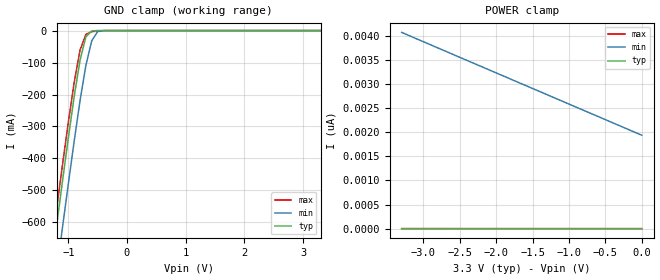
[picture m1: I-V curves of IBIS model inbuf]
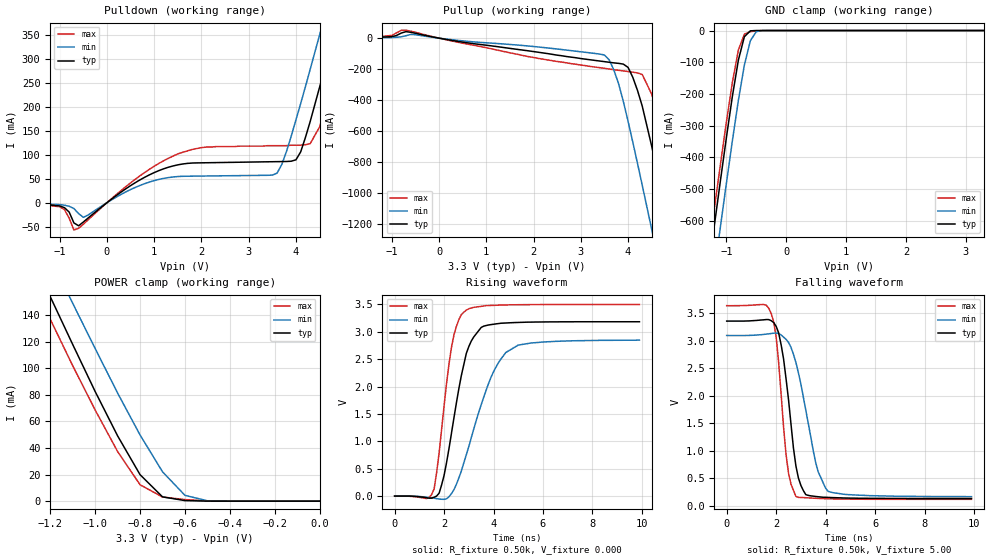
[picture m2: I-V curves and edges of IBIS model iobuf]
| IBIS file 43244k.ibs created by s2ibis2 version 1.0
| North Carolina State University Electronics Research Laboratory  1995
[IBIS ver]   2.1
[File name]   74fct3244.ibs
[File Rev]   0.1
[Date]   Wednesday, March 19, 1997
[Source]   IDT
[Notes]   1. Temp typ=25C, min=100C, max=0C 2. Ramp rates based on 500
   ohm load
[Copyright]   Copyright 1997, Integrated Device Technology, Inc.
|   Component IDT54/74FCT3245/A
[Component]   IDT54/74FCT3244/A
[Manufacturer]   Integrated Device Technology Inc.
[Package]
| Following package parameters are for D20-1(CDIP), P20-1(DPIP) packages
|[Package]
|| variable   typ   min   max
|R_pkg   40.00m   30.00m   50.00m
|L_pkg   7.00nH   4.00nH   10.00nH
|C_pkg   0.60pF   0.50pF   0.70pF
| Following package parameters are for SO20-6(EIAJ), SO20-2(SOIC) packages
|[Package]
|| variable   typ   min   max
|R_pkg   25.00m   20.00m   30.00m
|L_pkg   3.50nH   2.10nH   6.50nH
|C_pkg   0.40pF   0.35pF   0.60pF
| Following package parameters are for SO20-8(QSOP), SO20-7(SSOP) packages
| variable   typ   min   max
R_pkg   20.00m   15.00m   25.00m
L_pkg   3.00nH   2.00nH   4.00nH
C_pkg   0.30pF   0.26pF   0.34pF
[Pin]  signal_name   model_name   R_pin   L_pin   C_pin
1   1OEB   inbuf
2   1A1   inbuf
3   2Y4   iobuf
4   1A2   inbuf
5   2Y3   iobuf
6   1A3   inbuf
7   2Y2   iobuf
8   1A4   inbuf
9   2Y1   iobuf
10   GND   GND
11   2A1   inbuf
12   1Y4   iobuf
13   2A2   inbuf
14   1Y3   iobuf
15   2A3   inbuf
16   1Y2   iobuf
17   2A4   inbuf
18   1Y1   inbuf
19   2OEB   inbuf
20   VCC   POWER
| Models and submodels in the file (2): inbuf (Input), iobuf (I/O)
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| in   IN1   dummy_model
| oe   OE1   dummy_model
|   Model inbuf
[Model]   inbuf
Model_type   Input
Vinl =  0.800V
Vinh =  2.000V
C_comp   3.00pF   NA   NA
[Temperature Range]   25.00   100.00   0.000
[Voltage Range]   3.30V   3.00V   3.60V
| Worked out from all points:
|   GND clamp passes 1 mA (typ) near -0.60 V on its own axis
[GND_clamp]
| voltage   I(typ)   I(min)   I(max)
-3.3V     -3.672A    -3.825A    -3.588A
-1.3V     -753mA     -900mA     -698mA
-1.2V     -612mA     -758mA     -559mA
-1.1V     -473mA     -618mA     -422mA
-1V       -337mA     -481mA     -288mA
-900mV    -207mA     -347mA     -163mA
-800mV    -93.11mA   -220mA     -61.44mA
-700mV    -19.53mA   -109mA     -11.67mA
-600mV    -971uA     -32.12mA   -3.583mA
-500mV    -15.13uA   -3.312mA   -1.188mA
-400mV    -309nA     -162uA     -177uA
3.3V      308fA      2.133nA    132fA
[POWER_clamp]
| voltage   I(typ)   I(min)   I(max)
-3.3V     658fA      4.072nA    323fA
-2.5V     572fA      3.554nA    280fA
-2.2V     542fA      3.361nA    264fA
0V        309fA      1.939nA    148fA
|   Model iobuf
[Model]   iobuf
Model_type   I/O
Polarity   Non-Inverting
Enable   Active-High
Vinl =  0.800V
Vinh =  2.000V
C_comp   3.00pF   NA   NA
[Temperature Range]   25.00   100.00   0.000
[Voltage Range]   3.30V   3.00V   3.60V
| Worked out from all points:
|   slope of the pulldown table from 0 to 0.495 V, typ, clamps not added: 14 ohm
|   slope of the pullup table from 0 to 0.495 V, typ, clamps not added: 19.4 ohm
|   GND clamp passes 1 mA (typ) near -0.60 V on its own axis
|   POWER clamp passes 1 mA (typ) near -0.62 V on its own axis
|   rising waveform, R_fixture 0.50k, V_fixture 0.000: 20-80 % time 760ps typ, 1.23ns min, 561ps max; typ from 0 V to 3.18 V
|   falling waveform, R_fixture 0.50k, V_fixture 5.00: 20-80 % time 499ps typ, 767ps min, 403ps max; typ from 3.36 V to 0.128 V
[Pulldown]
| voltage   I(typ)   I(min)   I(max)
-3.3V     0A         -1mA       -1mA
-1V       -6.8mA     -4mA       -8.5mA
-700mV    -42.26mA   -12.2mA    -56.94mA
-500mV    -40.34mA   -30.59mA   -44.94mA
1.5V      78.96mA    54.58mA    102mA
3.5V      85.49mA    57.54mA    119mA
3.7V      85.8mA     79.63mA    119mA
4V        89.49mA    173mA      120mA
4.5V      241mA      350mA      158mA
4.9V      390mA      496mA      293mA
5.1V      466mA      569mA      365mA
6.6V      1.041A     1.126A     916mA
[Pullup]
| voltage   I(typ)   I(min)   I(max)
-3.3V     700uA      500uA      800uA
-700mV    42.09mA    15.79mA    51.26mA
3.5V      -152mA     -109mA     -195mA
3.7V      -160mA     -206mA     -204mA
4V        -189mA     -537mA     -216mA
4.3V      -439mA     -951mA     -235mA
4.5V      -698mA     -1.236A    -362mA
4.7V      -978mA     -1.524A    -557mA
4.9V      -1.263A    -1.815A    -819mA
5.1V      -1.552A    -2.107A    -1.098A
5.3V      -1.843A    -2.4A      -1.382A
6.6V      -3.751A    -4.318A    -3.265A
[GND_clamp]
| voltage   I(typ)   I(min)   I(max)
-3.3V     -3.672A    -3.825A    -3.588A
-1.3V     -753mA     -900mA     -698mA
-1.2V     -612mA     -758mA     -559mA
-1.1V     -473mA     -618mA     -422mA
-1V       -337mA     -481mA     -288mA
-900mV    -207mA     -347mA     -163mA
-800mV    -93.11mA   -220mA     -61.44mA
-700mV    -19.53mA   -109mA     -11.66mA
-600mV    -971uA     -32.12mA   -3.582mA
-500mV    -15.13uA   -3.312mA   -1.188mA
-400mV    -309nA     -162uA     -177uA
3.3V      307fA      540nA      120fA
[POWER_clamp]
| voltage   I(typ)   I(min)   I(max)
-3.3V     951mA      954mA      901mA
-1.3V     191mA      220mA      172mA
-1.2V     154mA      184mA      137mA
-1.1V     118mA      149mA      102mA
-1V       82.58mA    115mA      68.66mA
-900mV    49.17mA    81.42mA    37.36mA
-800mV    19.95mA    49.86mA    12.36mA
-700mV    3.23mA     22.14mA    3.104mA
-600mV    417uA      4.37mA     1.165mA
-500mV    2.462uA    264uA      211uA
0V        306fA      1.939nA    148fA
[Ramp]
| variable   typ   min   max
dV/dt_r   1.91/0.76n   1.71/1.23n   2.10/0.56n
dV/dt_f   1.93/0.50n   1.74/0.80n   2.11/0.39n
R_load = 0.50k
[Rising Waveform]
R_fixture = 0.50k
V_fixture = 0.000
| time   V(typ)   V(min)   V(max)
0s        0V         0V         0V
1.3ns     -31.47mV   -20.65mV   -46.2mV
1.6ns     -22.07mV   -39.47mV   134mV
1.9ns     202mV      -58.35mV   1.215V
2.3ns     1.149V     45.05mV    2.717V
2.6ns     1.966V     334mV      3.223V
2.9ns     2.605V     756mV      3.395V
3.5ns     3.078V     1.665V     3.464V
4.5ns     3.16V      2.622V     3.49V
9.9ns     3.183V     2.847V     3.498V
[Falling Waveform]
R_fixture = 0.50k
V_fixture = 5.00
| time   V(typ)   V(min)   V(max)
0s        3.358V     3.096V     3.639V
1.8ns     3.366V     3.132V     3.497V
2ns       3.263V     3.14V      3.07V
2.3ns     2.67V      3.066V     1.43V
2.5ns     1.93V      2.97V      590mV
2.8ns     719mV      2.604V     165mV
3.2ns     198mV      1.734V     142mV
3.6ns     165mV      779mV      132mV
4.1ns     148mV      258mV      122mV
9.9ns     128mV      162mV      113mV
